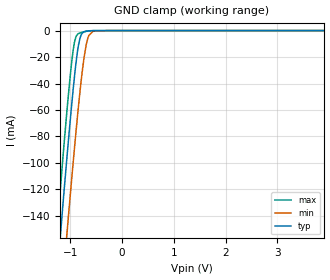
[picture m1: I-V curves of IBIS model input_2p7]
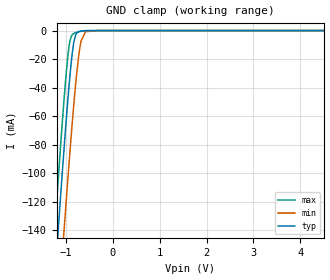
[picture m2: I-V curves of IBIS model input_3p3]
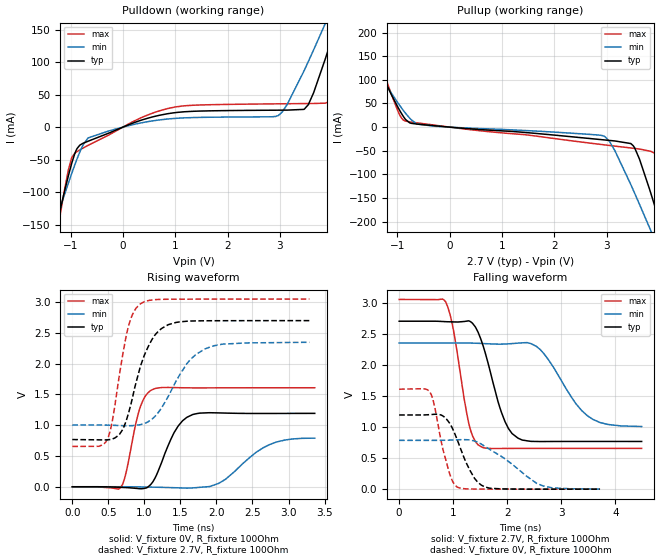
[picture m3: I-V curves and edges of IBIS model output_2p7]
|Texas Instruments Incorporated
| NA
| Marketing part#   Digital Voltage Range   Package-type   #pins
| ADS8912BRGE   1.65V-3.6V   QFN   24
[IBIS Ver]   4.1
[File name]   ads8912b.ibs
[File Rev]   1.0
[Date]   4/17/2015
[Source]
| Texas Instruments Incorporated.
| Analog-eLab Design Center, HPA
| 12500 TI Blvd
| Dallas, TX -75243
[Notes]   Revision History:
| Rev 1.0: 4/17/2015
| - Initial version of the model
| - Model generated from simulations in TISPICE
| - Model matched to SPICE simulation
| - C_comp although listed in numerical order of value are
|   obtained from varying PVT conditions. For PVT conditions for
|   each specific value refer the buffer description under
|   respective [Model]. IBIS model user is responsible for using
|   appropriate C_comp to simulate for Signal Integrity.
[Disclaimer]
| This model is designed as an aid for customers of Texas Instruments.
| TI and its licensors and suppliers make no warranties, either expressed
| or implied, with respect to this  model, including the warranties of
| merchantability or fitness for a particular purpose. The model is
| provided solely on an "as is" basis. The entire risk as to its quality
| and performance is with the customer.
[Copyright]
(C) Copyright 2015 Texas Instruments Incorporated.All rights reserved.
|   ADS8910RGE
[Component]   ADS8912BRGE
[Manufacturer]   TI
[Package]   |24 QFN   -  RGE package
|   typ   min   max
R_pkg   0.1   0.08   0.12
L_pkg   1.0nH   0.8nH   1.2nH
C_pkg   0.2pF   0.16pF   0.24pF
[Pin]  signal_name   model_name   R_pin   L_pin   C_pin
1   CONVST   INPUT   NA   NA   NA
2   RSTZ   INPUT   NA   NA   NA
3   REFIO   NC   NA   NA   NA
4   REFM_C   NC   NA   NA   NA
5   REFBUFOUT/REFP_C NC   NA   NA   NA
6   NC/TEST   NC   NA   NA   NA
7   REFP_F   NC   NA   NA   NA
8   REFM_F   NC   NA   NA   NA
9   AINP   NC   NA   NA   NA
10   AINM   NC   NA   NA   NA
11   GND   GND   NA   NA   NA
12   RVDD   POWER   NA   NA   NA
13   LDO-OUT   POWER   NA   NA   NA
14   AVDD   POWER   NA   NA   NA
15   GND   GND   NA   NA   NA
16   DVDD   POWER   NA   NA   NA
17   SDO-3   OUTPUT   NA   NA   NA
18   SDO-2   OUTPUT   NA   NA   NA
19   SDO-1   OUTPUT   NA   NA   NA
20   SDO-0   OUTPUT   NA   NA   NA
21   READY   OUTPUT   NA   NA   NA
22   SDI   INPUT   NA   NA   NA
23   SCLK   INPUT   NA   NA   NA
24   CSZ   INPUT   NA   NA   NA
|   Model Selectors
[Model Selector] INPUT
input_2p7   2.7V   digital Input
input_3p3   3.3V   digital Input
[Model Selector] OUTPUT
output_2p7   2.7V   digital Output
output_3p3   3.3V   digital Output
| Models and submodels in the file (4): input_2p7 (Input), input_3p3 (Input), output_2p7 (Output), output_3p3 (Output)
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|   input_2p7 Model
[Model]   input_2p7
Model_type   Input
Vinl = 0.81
Vinh = 1.89
|   typ   min   max
|   (nom PVT)   (fast PVT)   (slow PVT)
C_comp   3.663e-13   3.551e-13   3.771e-13
[Model spec]
|subparameter
Vinl   0.81   0.705   0.915
Vinh   1.89   1.645   2.135
| Where nom  PVT is Nominal Process, 2.7V, 27C
|   Fast PVT is Strong Process,  3.05V, -40C
|   Slow PVT is Weak Process,   2.35V, 125C
[Voltage Range]   2.7   2.35   3.05
|Junction Temperature
[Temperature Range]   27   125   -40
[Power Clamp Reference]   2.7   2.35   3.05
[GND Clamp Reference]   0   0   0
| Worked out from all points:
|   GND clamp passes 1 mA (typ) near -0.74 V on its own axis
[GND Clamp]
|   Voltage   I(typ)   I(min)   I(max)
-2.7V     -904.7mA   -955mA     -875.4mA
-1.431V   -268.3mA   -325.2mA   -233.6mA
-1.148V   -132.1mA   -189.9mA   -96.45mA
-1.075V   -98.54mA   -156.2mA   -63.31mA
-1.053V   -88.84mA   -146.3mA   -53.91mA
-949.3mV  -44.83mA   -100.1mA   -15.05mA
-897.4mV  -25.8mA    -78.1mA    -5.008mA
-845.8mV  -11.14mA   -57.27mA   -2.322mA
-789.4mV  -2.93mA    -36.49mA   -1.469mA
-695.5mV  -393uA     -10.6mA    -610.2uA
-561.5mV  -27.15uA   -493.5uA   -56.97uA
5.4V      0A         0A         0A
[POWER Clamp]
|   Voltage   I(typ)   I(min)   I(max)
-2.7V     0A         0A         0A
0V        0A         0A         0A
5.4V      0A         0A         0A
|   input_3p3 Model
[Model]   input_3p3
Model_type   Input
Vinl = 0.99
Vinh = 2.31
|   typ   min   max
|   (nom PVT)   (fast PVT)   (slow PVT)
C_comp   3.576e-13   3.444e-13   3.698e-13
[Model spec]
|subparameter
Vinl   0.99   0.9   1.08
Vinh   2.31   2.1   2.52
| Where nom  PVT is Nominal Process, 3.3V, 27C
|   Fast PVT is Strong Process,  3.6V, -40C
|   Slow PVT is Weak Process,   3V, 125C
[Voltage Range]   3.3   3   3.6
|Junction Temperature
[Temperature Range]   27   125   -40
[Power Clamp Reference]   3.3   3   3.6
[GND Clamp Reference]   0   0   0
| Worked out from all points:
|   GND clamp passes 1 mA (typ) near -0.74 V on its own axis
[GND Clamp]
|   Voltage   I(typ)   I(min)   I(max)
-3.3V     -1.21A     -1.257A    -1.182A
-1.614V   -358.4mA   -414.3mA   -324.6mA
-1.223V   -167.5mA   -225.3mA   -132mA
-1.209V   -161mA     -218.8mA   -125.4mA
-1.1V     -110.3mA   -168.1mA   -74.83mA
-1.047V   -86.17mA   -143.6mA   -51.34mA
-937.2mV  -40.15mA   -94.92mA   -11.89mA
-828.3mV  -7.641mA   -50.54mA   -1.986mA
-772.8mV  -1.927mA   -30.94mA   -1.288mA
-693mV    -376.3uA   -10.14mA   -592.9uA
-582mV    -43.61uA   -815.6uA   -92.29uA
6.6V      0A         0A         0A
[POWER Clamp]
|   Voltage   I(typ)   I(min)   I(max)
-3.3V     0A         0A         0A
0V        0A         0A         0A
6.6V      0A         0A         0A
|   output_2p7 Model
[Model]   output_2p7
Model_type   Output
Polarity   Non-Inverting
Vmeas = 1.65
Vref = 0
Cref = 20pF
Rref = 500
|   typ   min   max
|   (nom PVT)   (fast PVT)   (slow PVT)
C_comp   1.359e-12   1.328e-12   1.378e-12
| Where nom  PVT is Nominal Process, 2.7V, 27C
|   Fast PVT is Strong Process,  3.05V, -40C
|   Slow PVT is Weak Process,   2.35V, 125C
[Voltage Range]   2.7   2.35   3.05
|Junction Temperature
[Temperature Range]   27   125   -40
[Pullup Reference]   2.7   2.35   3.05
[Pulldown Reference]   0   0   0
[Power Clamp Reference]   2.7   2.35   3.05
[GND Clamp Reference]   0   0   0
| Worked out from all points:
|   slope of the pulldown table from 0 to 0.405 V, typ, clamps not added: 33.6 ohm
|   slope of the pullup table from 0 to 0.405 V, typ, clamps not added: 109 ohm
|   falling waveform, V_fixture 2.7V, R_fixture 100Ohm: 20-80 % time 378ps typ, 605ps min, 269ps max; typ from 2.7 V to 0.767 V
|   rising waveform, V_fixture 0V, R_fixture 100Ohm: 20-80 % time 266ps typ, 485ps min, 177ps max; typ from 0 V to 1.19 V
|   rising waveform, V_fixture 2.7V, R_fixture 100Ohm: 20-80 % time 299ps typ, 414ps min, 206ps max; typ from 0.767 V to 2.7 V
|   falling waveform, V_fixture 0V, R_fixture 100Ohm: 20-80 % time 353ps typ, 744ps min, 243ps max; typ from 1.19 V to 0 V
[Pulldown]
|   Voltage   I(typ)   I(min)   I(max)
-2.7V     -684.9mA   -513.4mA   -916.4mA
-1.474V   -225.5mA   -192.8mA   -272.7mA
-1.199V   -127.1mA   -123.8mA   -135mA
-975.1mV  -54.53mA   -70.25mA   -46.32mA
-667.3mV  -21.67mA   -16.63mA   -28.07mA
886.8mV   21.02mA    12.72mA    29.11mA
2.967V    26.07mA    17.68mA    35.83mA
3.467V    27.54mA    87.12mA    36.21mA
3.873V    105.6mA    159.8mA    36.83mA
4.092V    161mA      199.9mA    73.49mA
4.263V    204.8mA    231.1mA    130.1mA
5.4V      493.7mA    434.3mA    531.4mA
[Pullup]
|   Voltage   I(typ)   I(min)   I(max)
-2.7V     467.1mA    356.7mA    614.8mA
-1.379V   132.1mA    118mA      153.6mA
-988.9mV  41.43mA    50.83mA    33.15mA
-857.8mV  17.88mA    31mA       13.2mA
-270.1mV  2.733mA    1.734mA    3.928mA
2.921V    -26.69mA   -18.04mA   -36.99mA
3.461V    -34.69mA   -121.4mA   -44.06mA
3.821V    -131.6mA   -212.8mA   -50.6mA
3.943V    -175.1mA   -244.5mA   -56.76mA
4.132V    -244.1mA   -293.9mA   -123.8mA
4.367V    -331.2mA   -355.7mA   -239.5mA
5.4V      -720mA     -629.3mA   -778.3mA
[Ramp]
R_load = 100
|   typ   min   max
dV/dt_r   0.715687/2.64331e-10  0.470831/4.7653e-10   0.96524/1.77019e-10
dV/dt_f   1.15981/3.76756e-10   0.807974/6.05692e-10   1.43672/2.68308e-10
[Falling Waveform]
V_fixture = 2.7V
V_fixture_min = 2.35V
V_fixture_max = 3.05V
R_fixture = 100Ohm
|   Time   V(typ)   V(min)   V(max)
0s        2.7V       2.35V      3.05V
862ps     2.693V     2.35V      3.009V
1.004ns   2.689V     2.35V      2.562V
1.3ns     2.702V     2.349V     1.018V
1.51ns    2.417V     2.343V     686.5mV
1.894ns   1.234V     2.332V     654.2mV
2.198ns   821.3mV    2.348V     655.6mV
2.618ns   765.5mV    2.238V     655.8mV
3.482ns   767.6mV    1.182V     655.5mV
4.488ns   767.2mV    1.007V     655.5mV
[Rising Waveform]
V_fixture = 0V
V_fixture_min = 0V
V_fixture_max = 0V
R_fixture = 100Ohm
|   Time   V(typ)   V(min)   V(max)
0s        1.586nV    3.928nV    1.397nV
668ps     -9.296mV   352.7uV    -16.14mV
738ps     -13.13mV   120.8uV    189.4mV
948ps     -32.75mV   -2.351mV   1.31V
1.148ns   141.2mV    -7.108mV   1.596V
1.412ns   878.8mV    -15.31mV   1.611V
1.672ns   1.174V     -18.6mV    1.607V
2.03ns    1.2V       54.17mV    1.608V
2.74ns    1.191V     686.9mV    1.609V
3.364ns   1.192V     790mV      1.609V
[Rising Waveform]
V_fixture = 2.7V
V_fixture_min = 2.35V
V_fixture_max = 3.05V
R_fixture = 100Ohm
|   Time   V(typ)   V(min)   V(max)
0s        767mV      1.003V     655.5mV
484ps     762.2mV    1.001V     766.4mV
556ps     776.7mV    999.1mV    1.073V
652ps     847mV      995.1mV    1.803V
772ps     1.163V     992.1mV    2.574V
950ps     1.974V     1.011V     2.976V
1.242ns   2.574V     1.287V     3.046V
1.592ns   2.69V      2.004V     3.048V
1.84ns    2.697V     2.239V     3.049V
3.29ns    2.7V       2.348V     3.05V
[Falling Waveform]
V_fixture = 0V
V_fixture_min = 0V
V_fixture_max = 0V
R_fixture = 100Ohm
|   Time   V(typ)   V(min)   V(max)
0s        1.193V     784.7mV    1.607V
576ps     1.199V     784.5mV    1.551V
634ps     1.203V     784.5mV    1.412V
804ps     1.18V      785.6mV    663.8mV
912ps     1.087V     788mV      314mV
1.076ns   792.4mV    793.5mV    32.61mV
1.39ns    181.4mV    775mV      2.48mV
1.582ns   37.35mV    689.6mV    934.1uV
2.67ns    343.8uV    49.73mV    99.87uV
3.718ns   129.2uV    1.383mV    13.27uV
